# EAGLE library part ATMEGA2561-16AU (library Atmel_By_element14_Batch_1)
Microcontroller
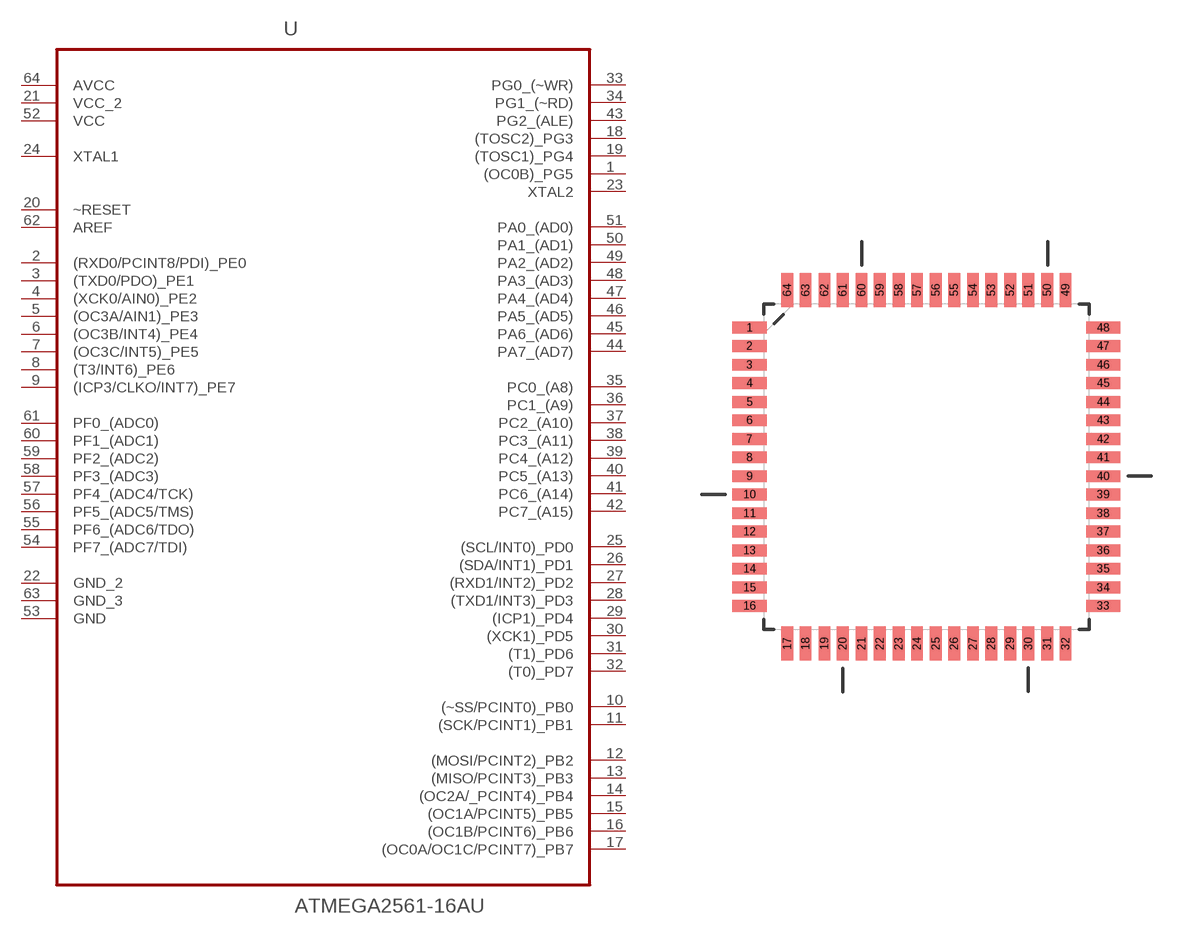
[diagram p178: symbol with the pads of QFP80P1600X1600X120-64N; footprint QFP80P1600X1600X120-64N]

Designator prefix U

## ATMEGA2561-16AU (DESCRIPTION: Microcontroller; MPN: ATMEGA2561-16AU; OC_FARNELL: 1288332; OC_NEWARK: 23M5053; PACKAGE: QFP-64; SUPPLIER: ATMEL)  [QFP80P1600X1600X120-64N]
1  (OC0B)_PG5
2  (RXD0/PCINT8/PDI)_PE0
3  (TXD0/PDO)_PE1
4  (XCK0/AIN0)_PE2
5  (OC3A/AIN1)_PE3
6  (OC3B/INT4)_PE4
7  (OC3C/INT5)_PE5
8  (T3/INT6)_PE6
9  (ICP3/CLKO/INT7)_PE7
10  (~SS/PCINT0)_PB0
11  (SCK/PCINT1)_PB1
12  (MOSI/PCINT2)_PB2
13  (MISO/PCINT3)_PB3
14  (OC2A/_PCINT4)_PB4
15  (OC1A/PCINT5)_PB5
16  (OC1B/PCINT6)_PB6
17  (OC0A/OC1C/PCINT7)_PB7
18  (TOSC2)_PG3
19  (TOSC1)_PG4
20  ~RESET  in
21  VCC_2  pwr
22  GND_2  pas
23  XTAL2  out
24  XTAL1  in
25  (SCL/INT0)_PD0
26  (SDA/INT1)_PD1
27  (RXD1/INT2)_PD2
28  (TXD1/INT3)_PD3
29  (ICP1)_PD4
30  (XCK1)_PD5
31  (T1)_PD6
32  (T0)_PD7
33  PG0_(~WR)
34  PG1_(~RD)
35  PC0_(A8)
36  PC1_(A9)
37  PC2_(A10)
38  PC3_(A11)
39  PC4_(A12)
40  PC5_(A13)
41  PC6_(A14)
42  PC7_(A15)
43  PG2_(ALE)
44  PA7_(AD7)
45  PA6_(AD6)
46  PA5_(AD5)
47  PA4_(AD4)
48  PA3_(AD3)
49  PA2_(AD2)
50  PA1_(AD1)
51  PA0_(AD0)
52  VCC  pwr
53  GND  pas
54  PF7_(ADC7/TDI)
55  PF6_(ADC6/TDO)
56  PF5_(ADC5/TMS)
57  PF4_(ADC4/TCK)
58  PF3_(ADC3)
59  PF2_(ADC2)
60  PF1_(ADC1)
61  PF0_(ADC0)
62  AREF  in
63  GND_3  pas
64  AVCC  pwr

## Footprint QFP80P1600X1600X120-64N (pad centres in mm)
smd 1.473 x 0.508: 1 -7.62,5.994; 2 -7.62,5.207; 3 -7.62,4.394; 4 -7.62,3.607; 5 -7.62,2.794; 6 -7.62,2.007; 7 -7.62,1.194; 8 -7.62,0.406; 9 -7.62,-0.406; 10 -7.62,-1.194; 11 -7.62,-2.007; 12 -7.62,-2.794; 13 -7.62,-3.607; 14 -7.62,-4.394; 15 -7.62,-5.207; 16 -7.62,-5.994; 33 7.62,-5.994; 34 7.62,-5.207; 35 7.62,-4.394; 36 7.62,-3.607; 37 7.62,-2.794; 38 7.62,-2.007; 39 7.62,-1.194; 40 7.62,-0.406; 41 7.62,0.406; 42 7.62,1.194; 43 7.62,2.007; 44 7.62,2.794; 45 7.62,3.607; 46 7.62,4.394; 47 7.62,5.207; 48 7.62,5.994
smd 0.508 x 1.473: 17 -5.994,-7.62; 18 -5.207,-7.62; 19 -4.394,-7.62; 20 -3.607,-7.62; 21 -2.794,-7.62; 22 -2.007,-7.62; 23 -1.194,-7.62; 24 -0.406,-7.62; 25 0.406,-7.62; 26 1.194,-7.62; 27 2.007,-7.62; 28 2.794,-7.62; 29 3.607,-7.62; 30 4.394,-7.62; 31 5.207,-7.62; 32 5.994,-7.62; 49 5.994,7.62; 50 5.207,7.62; 51 4.394,7.62; 52 3.607,7.62; 53 2.794,7.62; 54 2.007,7.62; 55 1.194,7.62; 56 0.406,7.62; 57 -0.406,7.62; 58 -1.194,7.62; 59 -2.007,7.62; 60 -2.794,7.62; 61 -3.607,7.62; 62 -4.394,7.62; 63 -5.207,7.62; 64 -5.994,7.62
